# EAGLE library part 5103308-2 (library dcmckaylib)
0.1" Header with polarizing key Mates with Ribbon Cable connector 1658621-2
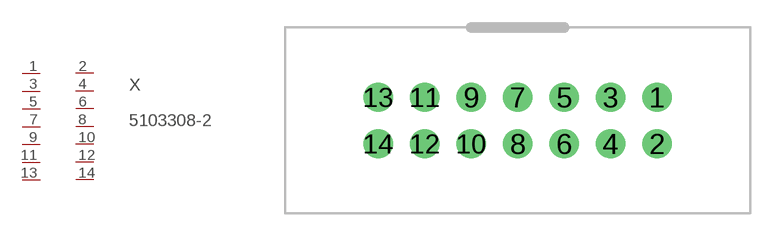
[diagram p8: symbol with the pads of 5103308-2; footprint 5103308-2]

Designator prefix X

## 5103308-2  [5103308-2]
1  P$1  pas
2  P$2  pas
3  P$3  pas
4  4  pas
5  5  pas
6  6  pas
7  7  pas
8  8  pas
9  9  pas
10  10  pas
11  11  pas
12  12  pas
13  13  pas
14  14  pas

## Footprint 5103308-2 (pad centres in mm)
drill 1.067: 1 7.62,1.27; 2 7.62,-1.27; 3 5.08,1.27; 4 5.08,-1.27; 5 2.54,1.27; 6 2.54,-1.27; 7 0,1.27; 8 0,-1.27; 9 -2.54,1.27; 10 -2.54,-1.27; 11 -5.08,1.27; 12 -5.08,-1.27; 13 -7.62,1.27; 14 -7.62,-1.27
